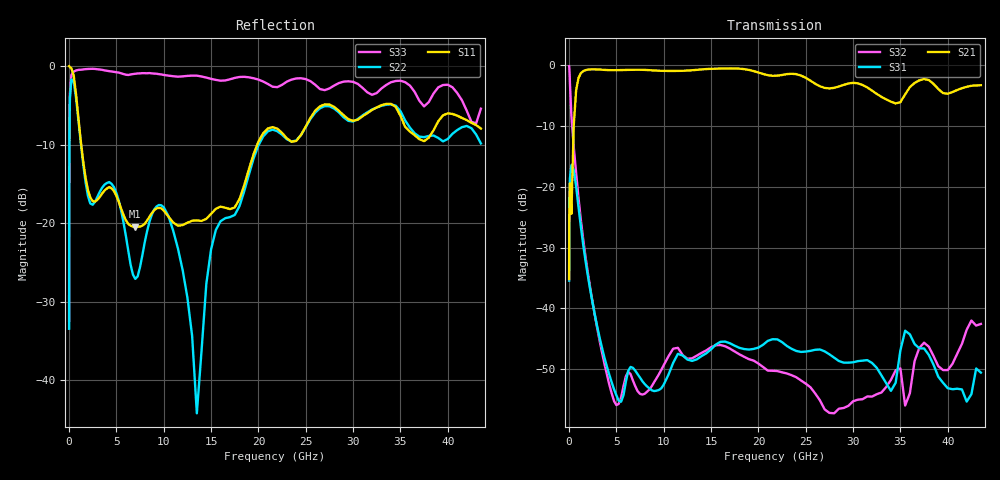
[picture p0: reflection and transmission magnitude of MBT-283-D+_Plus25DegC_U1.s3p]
! Model : MBT-283-D
! SerialNo: U1
! Port1: RF
! Port2: RF+DC
! Port3: DC
! Refer to datasheet on the assebly diagram
! Board loss is deducted using a THRU line
# Hz S dB R 50
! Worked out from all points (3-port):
!   117 points, 10 MHz to 43.5 GHz, reference 50 ohm
!   strongest paths, dB at 10 MHz, 5 GHz, 14.5 GHz, 29 GHz, 43.5 GHz:
!     S21: -35.2, -0.8, -0.6, -3.2, -3.3
!     S31: -35.4, -54.3, -47.4, -48.9, -50.6
!     S32: -0.1, -55.9, -46.9, -56.4, -42.6
!   lowest |S11| = -20.5 dB at 7 GHz (marker M1), VSWR 1.21, Z = 46.2 - j8.32 ohm
!   |S11| at or under -10 dB: 1.288 GHz to 19.88 GHz (18.59 GHz wide, 176 % of centre)
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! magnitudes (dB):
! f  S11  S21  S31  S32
! 10 MHz  0.0  -35.2  -35.4  -0.1
! 50 MHz  -0.1  -22.5  -22.5  -1.0
! 250 MHz  -0.3  -24.4  -16.4  -8.3
! 1 GHz  -6.7  -2.1  -23.3  -21.8
! 7 GHz  -20.5  -0.7  -50.3  -52.8
! 10.5 GHz  -19.2  -0.9  -50.9  -47.9
! 13.5 GHz  -19.6  -0.7  -48.4  -47.8
! 15.5 GHz  -18.2  -0.5  -46.0  -46.1
! 22 GHz  -8.0  -1.7  -45.1  -50.3
! 43.5 GHz  -7.9  -3.3  -50.6  -42.6
